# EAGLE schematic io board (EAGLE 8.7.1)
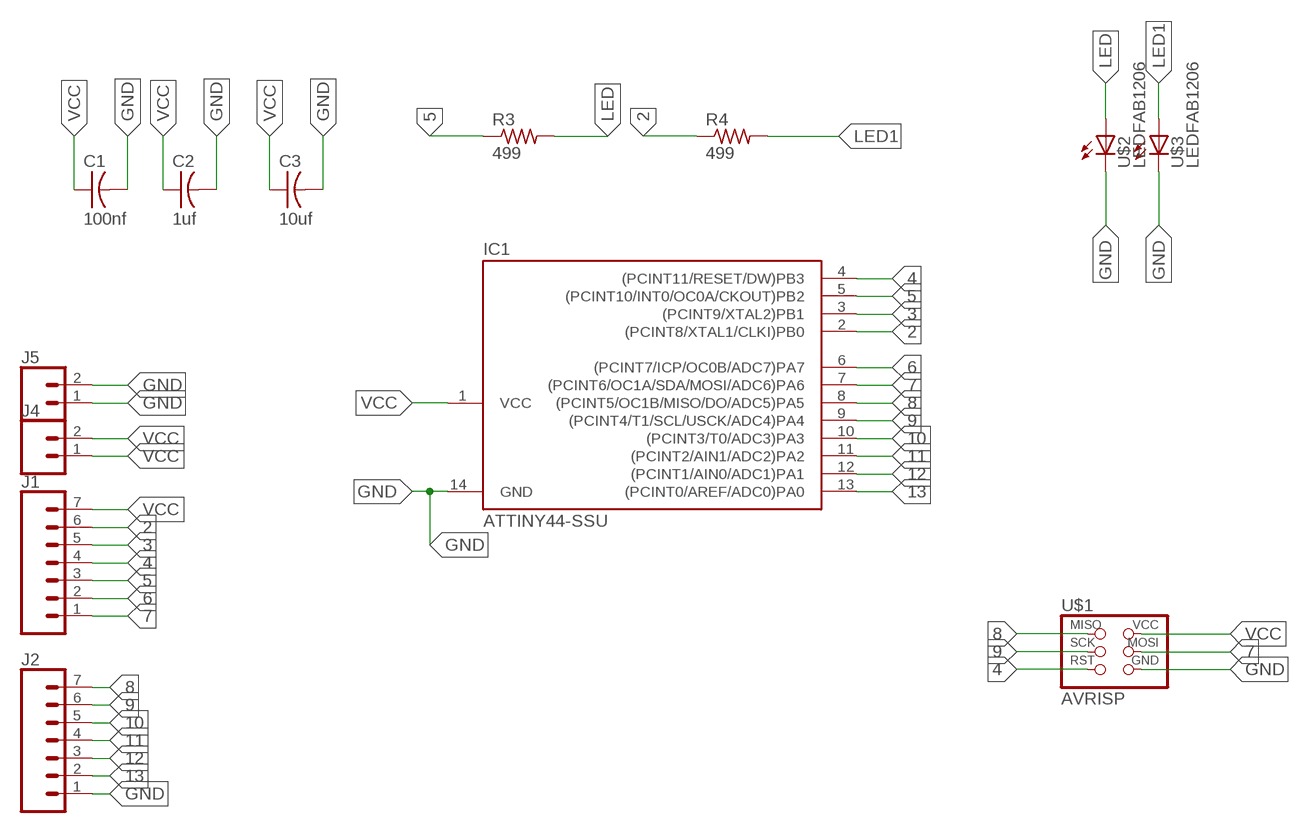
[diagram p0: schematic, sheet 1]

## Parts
C1  100nf  CAP-US1206FAB  [C1206FAB]
C2  1uf  CAP-US1206FAB  [C1206FAB]
C3  10uf  CAP-US1206FAB  [C1206FAB]
IC1  ATTINY44-SSU  [SOIC14]
J1  CONN_07  [1X07]
J2  CONN_07  [1X07]
J4  CONN_02  [1X02]
J5  CONN_02  [1X02]
R3  499  RES-US1206FAB  [R1206FAB]
R4  499  RES-US1206FAB  [R1206FAB]
U$1  AVRISP  [2X03]
U$2  LEDFAB1206  [LED1206FAB]
U$3  LEDFAB1206  [LED1206FAB]

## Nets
2: IC1.2((PCINT8/XTAL1/CLKI)PB0) J1.6 R4.1
3: IC1.3((PCINT9/XTAL2)PB1) J1.5
4: IC1.4((PCINT11/RESET/DW)PB3) J1.4 U$1.5(RST)
5: IC1.5((PCINT10/INT0/OC0A/CKOUT)PB2) J1.3 R3.1
6: IC1.6((PCINT7/ICP/OC0B/ADC7)PA7) J1.2
7: IC1.7((PCINT6/OC1A/SDA/MOSI/ADC6)PA6) J1.1 U$1.4(MOSI)
8: IC1.8((PCINT5/OC1B/MISO/DO/ADC5)PA5) J2.7 U$1.1(MISO)
9: IC1.9((PCINT4/T1/SCL/USCK/ADC4)PA4) J2.6 U$1.3(SCK)
10: IC1.10((PCINT3/T0/ADC3)PA3) J2.5
11: IC1.11((PCINT2/AIN1/ADC2)PA2) J2.4
12: IC1.12((PCINT1/AIN0/ADC1)PA1) J2.3
13: IC1.13((PCINT0/AREF/ADC0)PA0) J2.2
GND: C1.2 C2.2 C3.2 IC1.14(GND) J2.1 J5.1 J5.2 U$1.6(GND) U$2.2(C) U$3.2(C)
LED: R3.2 U$2.1(A)
LED1: R4.2 U$3.1(A)
VCC: C1.1 C2.1 C3.1 IC1.1(VCC) J1.7 J4.1 J4.2 U$1.2(VCC)

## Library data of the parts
C1-C3 = fab:CAP-US
IC1 = fab:ATTINY44
J1 J2 = SparkFun-Connectors:CONN_07: Multi connection point. Often used as Generic Header-pin footprint for 0.1 inch spaced/style header connections On any of the 0.1 inch spaced packages, you can populate with these: Break Away Headers - Straight (PRT-00116) Break Away Male Headers - Right Angle (PRT-00553) Female Headers (PRT-00115)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
J4 J5 = SparkFun-Connectors:CONN_02: Multi connection point. Often used as Generic Header-pin footprint for 0.1 inch spaced/style header connections
R3 R4 = fab:RES-US: Resistor (US Symbol)
U$1 = fab:AVRISP
U$2 U$3 = fab:LED: LED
